PROGRAM MAIN
VAR	
	nState: INT;	

	fbProductionConfigData : FB_ProductionConfigData;
	
	nTypeNum: DINT := 12345;
	stProductionConfig: ST_Config;
	
	stTestInfo: ST_TestParameter;
	
	sTestNum: STRING(7);
	sTimestamp: STRING;
	sTester: STRING;
	sResult: STRING;
END_VAR

CASE nState OF
	0:
		;
	1:// Get production config data
		IF fbProductionConfigData.GetConfig(nTypeNum:= nTypeNum, stConfig=> stProductionConfig) THEN
			IF fbProductionConfigData.bError THEN
				nState := 255;
			ELSE
				nState := 2;
			END_IF			
		END_IF
	2:// Produce product
	
		//.... Add here your production routine based on the config data
	
		nState := 3;
	3:// Get test parameter
		IF fbProductionConfigData.GetTestParameter(nTypeNum:= nTypeNum, sTestNum=> sTestNum, stTestPara=> stTestInfo) THEN
			IF fbProductionConfigData.bError THEN
				nState := 255;
			ELSE
				nState := 4;
			END_IF			
		END_IF 
	4:// Test your product
	
		//.... Add here your test routine based on the test parameter
		
		sTimestamp := '2017-01-20-12:13';
		sTester := 'Mustermann';
		sResult := 'OK';
		
		nState := 5;
	5:// Save test result
		IF fbProductionConfigData.AddTestEntry(
				sTestNum:= sTestNum, 
				nTypeNum:= nTypeNum, 
				sTimestamp:=sTimestamp, 
				sTester:= sTester, 
				sResult:= sResult) THEN
			IF fbProductionConfigData.bError THEN
				nState := 255;
			ELSE
				nState := 0;
			END_IF			
		END_IF
	255:
		;
END_CASE

END_PROGRAM
